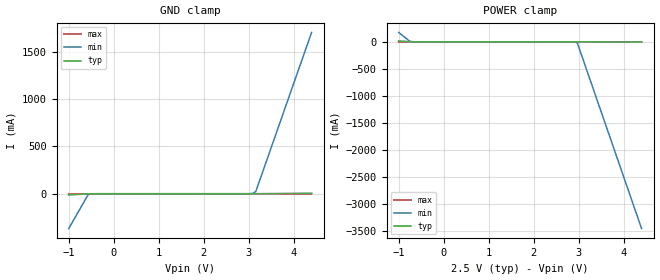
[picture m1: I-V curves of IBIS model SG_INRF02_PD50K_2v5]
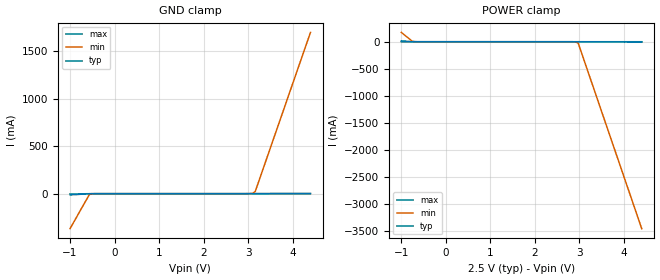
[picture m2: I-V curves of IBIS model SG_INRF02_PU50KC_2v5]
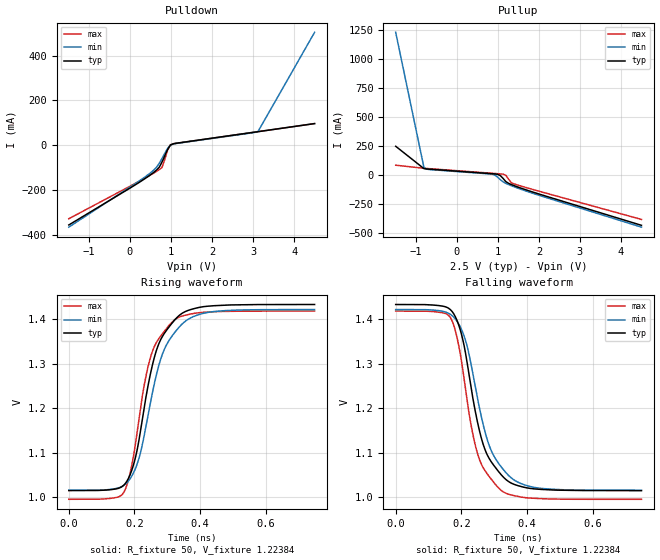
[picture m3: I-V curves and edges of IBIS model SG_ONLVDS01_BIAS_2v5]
|   This file is an IBIS representation of the   |
|   Integrated Device Technology , Inc.   |
|   ICS854S006I   |
|   LOW SKEW, 1-TO-6, DIFFERENTIAL-TO-LVDS FANOUT BUFFER   |
[IBIS Ver]   4.1
[File name]   854s006i.ibs
[File Rev]   1.0
[Date]   22 Jan 2010
[Source]   Originated at Integrated Device Technology, Inc.
[Disclaimer]
IDT hereby grants the user of this IBIS model a non-exclusive,
nontransferable license to use this IBIS model under the following terms.
Before using this IBIS model, the user should read this license.
If the user does not accept these terms,  the IBIS model should be
returned to IDT within 30 days.
   The user is granted this license only to use the IBIS model and
is not granted rights to sell, load, rent, lease or license the IBIS
model in whole or in part, or in modified form to anyone other than
user. User may modify the IBIS model to suit its specific
applications but rights to derivative works and such modifications
shall belong to IDT.
   This IBIS model is provided on an "AS IS" basis and IDT makes
absolutely no warranty with respect to the information contained
herein. IDT DISCLAIMS AND CUSTOMER WAIVES ALL WARRANTIES, EXPRESS
OR IMPLIED, INCLUDING WARRANTIES OF MERCHANTABILITY OR FITNESS FOR
A PARTICULAR PURPOSE. The entire risk as to quality and performance
is with the Customer. ACCORDINGLY, IN NO EVENT SHALL THE COMPANY BE
LIABLE FOR ANY DAMAGES, WHETHER IN CONTRACT OR TORT,INCLUDING ANY
LOST PROFITS OR OTHER INCIDENTAL, CONSEQUENTIAL, EXEMPLARY, OR
PUNITIVE DAMAGES ARISING OUT OF THE USE OR APPLICATION OF THE IBIS
model provided in this package. Further, IDT reserves the right to
make changes without notice to any product herein to improve
reliability, function, or design. IDT does not convey any license
under patent rights or any other intellectual property rights,
including those of third parties.
   IDT is not obligated to provide maintenance or support
for the licensed IBIS model.
[Copyright]   Copyright 2010 by Integrated Device Technology, Inc.
[Component]   ICS854S006GI
[Manufacturer] Integrated Device Technology, Inc.
[Package]
|TSSOP 24 Lead
|   typ   min   max
R_pkg   60.65m   52.4m   68.9m
L_pkg   1.989nH   1.431nH   2.547nH
C_pkg   0.314pF   0.254pF   0.374pF
[Pin] signal_name  model_name   R_pin   L_pin   C_pin
1   nCLK   SG_INRF02_PD50K   68.9m   2.547n   0.374p
2   CLK   SG_INRF02_PU50KC   65.6m   2.323n   0.350p
3   VDD   POWER   62.3m   2.100n   0.326p
4   VDDO   POWER   59.0m   1.877n   0.302p
5   QO   SG_ONLVDS01_BIAS   55.7m   1.654n   0.278p
6   nQ0   SG_ONLVDS01_BIAS   52.4m   1.431n   0.254p
7   GND   GND   52.4m   1.431n   0.254p
8   Q1   SG_ONLVDS01_BIAS   55.7m   1.654n   0.278p
9   nQ1   SG_ONLVDS01_BIAS   59.0m   1.877n   0.302p
10   VDDO   POWER   62.3m   2.100n   0.326p
11   Q2   SG_ONLVDS01_BIAS   65.6m   2.323n   0.350p
12   nQ2   SG_ONLVDS01_BIAS   68.9m   2.547n   0.374p
13   Q3   SG_ONLVDS01_BIAS   68.9m   2.547n   0.374p
14   nQ3   SG_ONLVDS01_BIAS   65.6m   2.323n   0.350p
15   VDDO   POWER   62.3m   2.100n   0.326p
16   Q4   SG_ONLVDS01_BIAS   59.0m   1.877n   0.302p
17   nQ4   SG_ONLVDS01_BIAS   55.7m   1.654n   0.278p
18   GND   GND   52.4m   1.431n   0.254p
19   Q5   SG_ONLVDS01_BIAS   52.4m   1.431n   0.254p
20   nQ5   SG_ONLVDS01_BIAS   55.7m   1.654n   0.278p
21   VDDO   POWER   59.0m   1.877n   0.302p
22   VDD   POWER   62.3m   2.100n   0.326p
23   GND   GND   65.6m   2.323n   0.350p
24   GND   GND   68.9m   2.547n   0.374p
[Diff Pin]  inv_pin  vdiff tdelay_typ tdelay_min  tdelay_max
2   1   0.15  NA   NA   NA
5   6   NA   0   0   0
8   9   NA   0   0   0
11   12   NA   0   0   0
13   14   NA   0   0   0
16   17   NA   0   0   0
19   20   NA   0   0   0
[Model Selector] SG_INRF02_PD50K
SG_INRF02_PD50K_2v5  Buffer selection for 2v5
SG_INRF02_PD50K_3v3  Buffer selection for 3v3
[Model Selector] SG_INRF02_PU50KC
SG_INRF02_PU50KC_2v5  Buffer selection for 2v5
SG_INRF02_PU50KC_3v3  Buffer selection for 3v3
[Model Selector] SG_ONLVDS01_BIAS
SG_ONLVDS01_BIAS_2v5  Buffer selection for 2v5
SG_ONLVDS01_BIAS_3v3  Buffer selection for 3v3
| Models and submodels in the file (6): SG_INRF02_PD50K_2v5 (Input), SG_INRF02_PU50KC_2v5 (Input), SG_ONLVDS01_BIAS_2v5 (Output), SG_INRF02_PD50K_3v3 (Input), SG_INRF02_PU50KC_3v3 (Input), SG_ONLVDS01_BIAS_3v3 (Output)
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[Model] SG_INRF02_PD50K_2v5
Model_type   Input
Polarity   Non-Inverting
Vinl = 0.7V
Vinh = 1.7V
|   typ   min   max
C_comp   2pF   1.5pF   2.5pF
|   typ   min   max
[Voltage range]   2.5V   2.375V   2.625V
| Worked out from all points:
|   GND clamp passes 1 mA (typ) near -0.58 V on its own axis
|   POWER clamp passes 1 mA (typ) near -0.75 V on its own axis
[GND_clamp]
|Voltage   I (typ)   I (min)   I (max)
-999mV    -13.4mA    -368.6mA   -3.626mA
-564.6mV  -601.6uA   -8.535mA   -255.2uA
-502.5mV  -178.6uA   -1.359mA   -57.43uA
2.973V    59.37uA    225.5uA    55.12uA
3.097V    80.54uA    3.606mA    57.43uA
3.159V    147.1uA    22.31mA    58.65uA
4.4V      5.221mA    1.703A     95.15uA
[Power_clamp]
|Voltage   I (typ)   I (min)   I (max)
-999mV    16.89mA    173.7mA    1.102mA
-750.8mV  768uA      8.333mA    137.3uA
-688.7mV  227uA      1.485mA    75.81uA
2.787V    -5.908uA   -116.4uA   -2.995uA
2.911V    -23.44uA   -3.554mA   -5.302uA
2.973V    -93.35uA   -23.91mA   -6.559uA
4.4V      -5.763mA   -3.459A    -69.61uA
[Model] SG_INRF02_PU50KC_2v5
Model_type   Input
Polarity   Non-Inverting
Vinl = 0.7V
Vinh = 1.7V
|   typ   min   max
C_comp   2pF   1.5pF   2.5pF
|   typ   min   max
[Voltage range]   2.5V   2.375V   2.625V
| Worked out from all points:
|   GND clamp passes 1 mA (typ) near -0.58 V on its own axis
|   POWER clamp passes 1 mA (typ) near -0.76 V on its own axis
[GND_clamp]
|Voltage   I (typ)   I (min)   I (max)
-999mV    -13.45mA   -368.7mA   -3.675mA
-564.6mV  -651uA     -8.583mA   -303.9uA
-502.5mV  -228uA     -1.408mA   -106.1uA
2.973V    9.717uA    128.4uA    6.447uA
3.097V    23.55uA    3.294mA    8.752uA
3.159V    65.49uA    21.84mA    9.944uA
4.4V      3.728mA    1.699A     41.22uA
[Power_clamp]
|Voltage   I (typ)   I (min)   I (max)
-999mV    16.01mA    172.7mA    690.8uA
-750.8mV  558.7uA    7.945mA    57.6uA
-688.7mV  119uA      1.251mA    21.36uA
2.787V    -55.29uA   -164.9uA   -51.67uA
2.911V    -72.82uA   -3.603mA   -53.98uA
2.973V    -142.7uA   -23.96mA   -55.24uA
4.4V      -5.813mA   -3.459A    -118.3uA
[Model] SG_ONLVDS01_BIAS_2v5
Model_type   Output
Polarity   Non-Inverting
|   typ   min   max
C_comp   2pF   1.5pF   2.5pF
Vmeas = 1.22V
Rref = 50
Cref = 0
Vref = 1.22V
|   typ   min   max
[Voltage range]   2.5V   2.375V   2.625V
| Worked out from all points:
|   slope of the pulldown table from 0 to 0.375 V, typ, clamps not added: 8.63 ohm
|   slope of the pullup table from 0 to 0.375 V, typ, clamps not added: 38.7 ohm
|   rising waveform, R_fixture 50, V_fixture 1.22384: 20-80 % time 71ps typ, 79.1ps min, 63.9ps max; typ from 1.01 V to 1.43 V
|   falling waveform, R_fixture 50, V_fixture 1.22384: 20-80 % time 71ps typ, 79.1ps min, 63.9ps max; typ from 1.43 V to 1.01 V
[Pulldown]
|Voltage   I (typ)   I (min)   I (max)
-1.49V    -353.8mA   -363.5mA   -326.1mA
300.1mV   -155.6mA   -148.9mA   -151.7mA
575.5mV   -120.5mA   -110.2mA   -123.3mA
644.4mV   -110.2mA   -97.82mA   -115.8mA
713.2mV   -97.35mA   -80.01mA   -107.8mA
782.1mV   -73.51mA   -57.71mA   -97.8mA
919.8mV   -17.01mA   -12.41mA   -19.62mA
988.6mV   1.882mA    1.482mA    3.446mA
1.126V    9.58mA     8.547mA    9.416mA
3.123V    61.2mA     62.29mA    61.4mA
4.5V      97.12mA    503.1mA    97.26mA
[Pullup]
|Voltage   I (typ)   I (min)   I (max)
-1.49V    250.5mA    1.232A     87.1mA
-801.5mV  57.94mA    66.92mA    60.88mA
-732.6mV  54.96mA    52.82mA    59.06mA
-663.8mV  53.1mA     49.73mA    57.26mA
850.9mV   13.95mA    9.808mA    17.83mA
919.8mV   12.09mA    2.974mA    16.03mA
988.6mV   9.219mA    -13.96mA   14.24mA
1.057V    -1.417mA   -36.8mA    12.43mA
1.195V    -54.31mA   -69.24mA   65.99uA
1.333V    -80.07mA   -90.09mA   -65.47mA
1.539V    -107.4mA   -117.3mA   -89.81mA
4.5V      -430.8mA   -446.6mA   -380.1mA
[Ramp]
|   typ   min   max
dV/dt_r   0.334/0.124n   0.324/0.136n   0.338/0.113n
dV/dt_f   0.334/0.124n   0.324/0.136n   0.338/0.113n
R_load =   50.0000
[Rising Waveform]
R_fixture = 50
V_fixture   =1.22384  |Vcc_typ
V_fixture_min=1.2185   |Vcc_min
V_fixture_max=1.20667  |Vcc_max
C_fixture = 0.0p
| Time   typ   min   max
0s        1.015V     1.015V     995.2mV
167.4ps   1.027V     1.027V     1.011V
185.4ps   1.048V     1.04V      1.05V
203.5ps   1.09V      1.065V     1.121V
226.7ps   1.187V     1.127V     1.239V
249.2ps   1.279V     1.214V     1.315V
283ps     1.358V     1.317V     1.365V
322.8ps   1.398V     1.37V      1.399V
425.7ps   1.429V     1.415V     1.416V
749.2ps   1.433V     1.421V     1.418V
[Falling Waveform]
R_fixture = 50
V_fixture   =1.22384  |Vcc_typ
V_fixture_min=1.2185   |Vcc_min
V_fixture_max=1.20667  |Vcc_max
C_fixture = 0.0p
| Time   typ   min   max
0s        1.433V     1.422V     1.418V
167.4ps   1.421V     1.41V      1.403V
185.4ps   1.4V       1.397V     1.364V
203.5ps   1.358V     1.372V     1.292V
226.7ps   1.26V      1.31V      1.175V
249.2ps   1.169V     1.223V     1.099V
283ps     1.09V      1.12V      1.049V
322.8ps   1.049V     1.067V     1.015V
425.7ps   1.018V     1.022V     997.5mV
749.2ps   1.015V     1.016V     995.2mV
